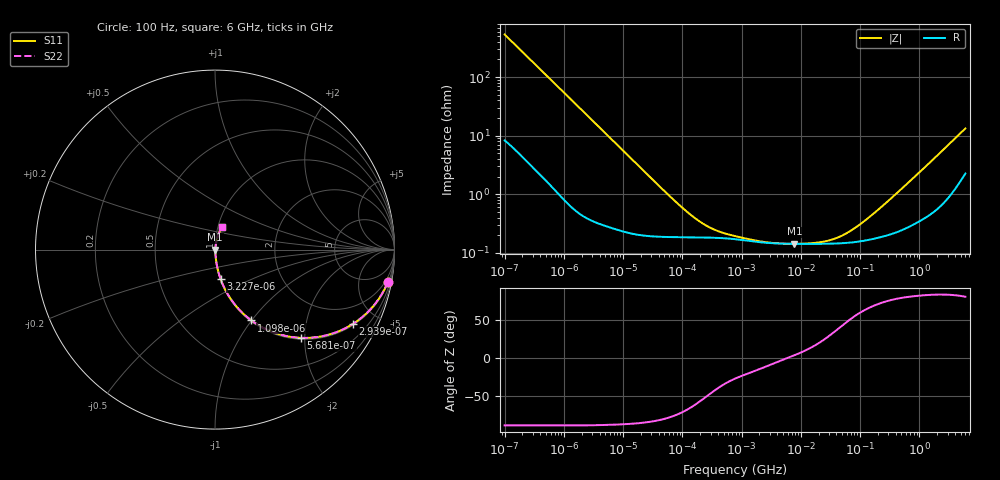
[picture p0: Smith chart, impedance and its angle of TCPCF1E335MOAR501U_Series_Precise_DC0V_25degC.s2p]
! TCPCF1E335MOAR501U Polymer Tantalum Capacitor Sparameter Model
! Model Generated by Samsung Electro-Mechanics
! Samsung Sparameter Version 5.0
! Date : Oct-10-2024
! Products : Polymer Tantalum Capacitor
! Characteristics :
!  Nominal Capacitance = 3.3uF
!  Capacitance Tolerance = +/-20%
!  ESR = 500 mohm max at 100kHz
!  Rated Voltage = 25Vdc
!  Size = 0805(unit:inch), 2012(unit:mm)
!  Length = 2.00+/-0.20mm
!  Width = 1.25+/-0.20mm
!  Thickness = 0.70+/-0.10mm
!  Lineup = Conductive Polymer Type
!  Feature = PCF
!  Measurement Temperature : 25degC.
!  DC bias Value = 0V
!  Frequency : 100Hz ~ 6GHz
! External Node Assignments :
!  1  o---||---o  2
# MHz S RI R 50.0
! Freq.  Real(S11)  Im(S11)  Real(S12)  Im(S12)  Real(S21)  Im(S21)  Real(S22)  Im(S22)
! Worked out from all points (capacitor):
!   300 points, 100 Hz to 6 GHz, reference 50 ohm
!   read as one part in series: C = 2.97 uF near 106.2 Hz
!   lowest |Z| = 143 mohm at 7.773 MHz (marker M1)
!   series resonance near 6.18 MHz, so ESL is about 220 pH
!   S11 on the Smith chart (normalised r, x): 100 Hz: 1, -11; 293.9 Hz: 1.06, -3.68; 568.1 Hz: 1.03, -1.92; 1.098 kHz: 1.01, -1.00; 3.227 kHz: 1.01, -0.34; 6 GHz: 1.05, +0.26
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0.0001  0.9636 -0.1797  0.0364 0.1797  0.0364 0.1797  0.9636 -0.1797
0.0001820283  0.8936 -0.3003  0.1064 0.3003  0.1064 0.3003  0.8936 -0.3003
0.0002939341  0.7687 -0.4137  0.2313 0.4137  0.2313 0.4137  0.7687 -0.4137
0.000568071  0.4797 -0.4919  0.5203 0.4919  0.5203 0.4919  0.4797 -0.4919
0.001097881  0.203 -0.3949  0.797 0.3949  0.797 0.3949  0.203 -0.3949
0.001998454  0.0738 -0.2536  0.9262 0.2536  0.9262 0.2536  0.0738 -0.2536
0.003227047  0.0314 -0.1648  0.9686 0.1648  0.9686 0.1648  0.0314 -0.1648
0.008933904  0.00621 -0.0616  0.9938 0.0616  0.9938 0.0616  0.00621 -0.0616
0.03993819  0.00208 -0.0139  0.9979 0.0139  0.9979 0.0139  0.00208 -0.0139
0.1041383  0.00188 -0.00538  0.9981 0.00538  0.9981 0.00538  0.00188 -0.00538
0.2012627  0.00185 -0.00283  0.9982 0.00283  0.9982 0.00283  0.00185 -0.00283
0.366355  0.00181 -0.00163  0.9982 0.00163  0.9982 0.00163  0.00181 -0.00163
0.7981464  0.00171 -0.000875  0.9983 0.000875  0.9983 0.000875  0.00171 -0.000875
2.644602  0.00149 -0.000298  0.9985 0.000298  0.9985 0.000298  0.00149 -0.000298
7.773385  0.00143 7.74e-05  0.9986 -7.74e-05  0.9986 -7.74e-05  0.00143 7.74e-05
15.95059  0.00143 0.000369  0.9986 -0.000369  0.9986 -0.000369  0.00143 0.000369
32.7298  0.00144 0.000858  0.9986 -0.000858  0.9986 -0.000858  0.00144 0.000858
59.57749  0.00149 0.00159  0.9985 -0.00159  0.9985 -0.00159  0.00149 0.00159
122.25  0.00164 0.0032  0.9984 -0.0032  0.9984 -0.0032  0.00164 0.0032
318.7652  0.00212 0.0079  0.9979 -0.0079  0.9979 -0.0079  0.00212 0.0079
1810.813  0.00678 0.0408  0.9932 -0.0408  0.9932 -0.0408  0.00678 0.0408
6000  0.0381 0.1236  0.9619 -0.1236  0.9619 -0.1236  0.0381 0.1236
